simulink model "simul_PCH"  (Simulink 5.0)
settings: Solver=ode4  StartTime=0.0  StopTime=20.0  FixedStep=0.01  RelTol=1e-3
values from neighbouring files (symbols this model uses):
  citatel_simul = [cit2 cit1 cit0]    [kvadaprox1.m]    (also in kvadaprox2.m; linaprox1.m = [cit1 cit0]; linaprox2.m; smith.m)
  D = uicontrol(gcf,   'Style','edit',   'ForegroundColor','black',   'BackgroundColor',[1 1 1],   'String',num2str(D),   'Position',[100 18 80 20],   'CallBack',['D=str2num(get(D,''String''));'])    [sus1.m]    (also in sus2.m = uicontrol(gcf,   'Style','edit',   'ForegroundColor','black')
  menovatel_simul = [men3 men2 men1 men0]    [kvadaprox1.m]    (also in kvadaprox2.m = [men4 men3 men2 men1 men0]; linaprox1.m = [men2 men1 men0]; linaprox2.m; smith.m)
  T = uicontrol(gcf,   'Style','edit',   'ForegroundColor','black',   'BackgroundColor',[1 1 1],   'String',num2str(T),   'Position',[100 40 80 20],   'CallBack',['T=str2num(get(T,''String''));'])    [sus1.m]    (also in sus2.m = uicontrol(gcf,   'Style','edit',   'ForegroundColor','black')
  Z = uicontrol(gcf,   'Style','edit',   'ForegroundColor','black',   'BackgroundColor',[1 1 1],   'String',num2str(Z),   'Position',[100 62 80 20],   'CallBack',['Z=str2num(get(Z,''String''));'])    [sus1.m]    (also in sus2.m = uicontrol(gcf,   'Style','edit',   'ForegroundColor','black')

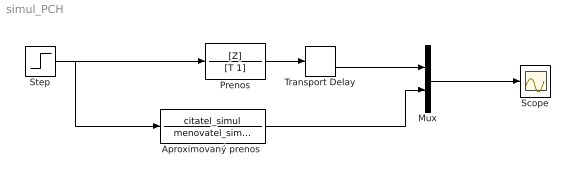
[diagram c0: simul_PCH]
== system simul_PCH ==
  "Aproximovaný prenos " : TransferFcn  Numerator=citatel_simul  Denominator=menovatel_simul
  Mux : Mux  Inputs=2
  Prenos : TransferFcn  Numerator=[Z]  Denominator=[T 1]
  Scope : Scope
  Step : Step  Time=0  SampleTime=0
  Transport Delay : TransportDelay  DelayTime=D
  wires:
  Step/1 -> Prenos/1, "Aproximovaný prenos "/1
  Mux/1 -> Scope/1
  "Aproximovaný prenos "/1 -> Mux/2
  Prenos/1 -> Transport Delay/1
  Transport Delay/1 -> Mux/1
